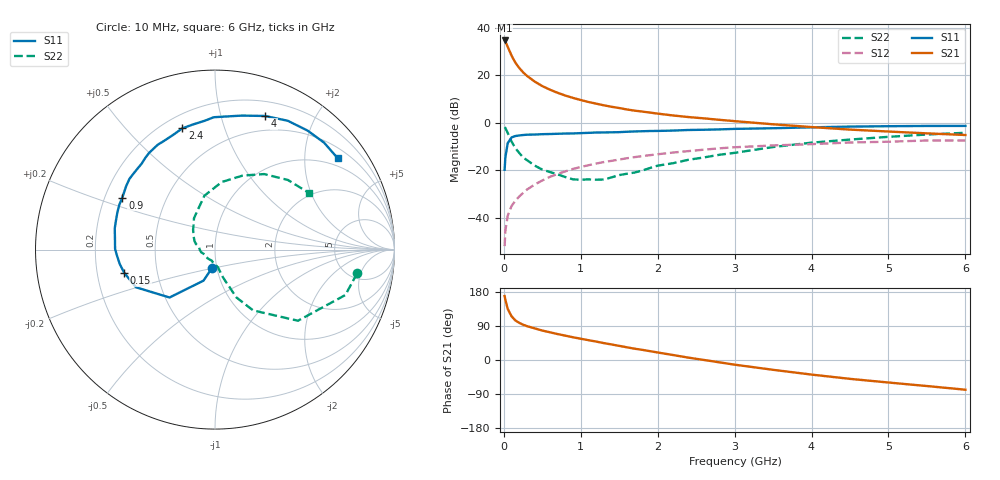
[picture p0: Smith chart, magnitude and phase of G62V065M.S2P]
! SIEMENS Small Signal Semiconductors
! BFG193
! Si NPN RF Bipolar Junction Transistor in SOT223
! VCE = 2 V  IC = 65 mA
! Common Emitter S-Parameters:  August  1996
# GHz  S  MA  R  50
!  f  S11  S21  S12  S22
! GHz  MAG  ANG  MAG  ANG  MAG  ANG  MAG  ANG
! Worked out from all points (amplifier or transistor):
!   36 points, 10 MHz to 6 GHz, reference 50 ohm
!   highest |S21| = 34.6 dB at 10 MHz (marker M1)
!   |S21| within 3 dB of that: start of sweep to 55.13 MHz
!   unconditionally stable (mu >= 1): start of sweep to 13.56 MHz; 234 MHz to 2.78 GHz
!   at 250 MHz: K = 1.02, MAG = 24.6 dB, |S12| = -29.6 dB
!   at 1.4 GHz: K = 1.09, MAG = 9.6 dB, |S12| = -16.1 dB
!   at 6 GHz: K = 0.97, MSG = 1.1 dB, |S12| = -7.5 dB
!   S11 on the Smith chart (normalised r, x): 10 MHz: 0.95, -0.19; 150 MHz: 0.32, -0.11; 900 MHz: 0.27, +0.24; 2.4 GHz: 0.28, +0.73; 4 GHz: 0.34, +1.39; 6 GHz: 0.76, +2.84
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0.01  0.1018 -98.6  53.74 168.8  0.0025 76.4  0.8026 -9.5
0.02  0.1848 -110.4  50.88 159.0  0.0053 75.8  0.7693 -19.2
0.05  0.3679 -133.5  39.77 135.1  0.0109 65.1  0.6089 -40.6
0.1  0.4878 -154.5  25.82 115.4  0.0175 64.1  0.4 -57.9
0.15  0.5219 -165.6  18.32 104.3  0.0227 64.6  0.2902 -66.1
0.2  0.5368 -171.4  14.21 98.1  0.0278 67.3  0.2297 -68.5
0.25  0.5479 -176.8  11.48 93.2  0.033 67.9  0.1854 -71.7
0.3  0.5567 179.6  9.672 89.4  0.0389 68.9  0.1622 -73.8
0.4  0.5608 173.7  7.328 83.5  0.0495 69.1  0.1248 -77.1
0.5  0.571 168.0  5.88 77.7  0.0605 68.1  0.1023 -79.9
0.6  0.5754 163.4  4.927 73.1  0.0722 66.9  0.091 -84.6
0.7  0.5823 159.0  4.24 68.4  0.083 65.6  0.0812 -91.7
0.9  0.5921 150.7  3.314 60.0  0.106 61.6  0.0638 -107.1
1.1  0.6089 144.3  2.718 52.3  0.1266 57.9  0.0638 -129.2
1.6  0.6424 127.1  1.892 33.5  0.1777 46.4  0.0838 -178.1
2.2  0.6798 110.2  1.414 13.1  0.2344 32.2  0.1397 148.4
2.4  0.6995 105.1  1.31 6.2  0.2513 27.8  0.1651 137.7
3.5  0.7614 78.7  0.922 -25.9  0.3306 -0.2  0.3061 101.1
4  0.7953 69.4  0.806 -38.5  0.3525 -10.1  0.3784 84.3
4.5  0.8245 60.5  0.713 -49.8  0.381 -20.4  0.4398 69.6
5.5  0.8511 44.4  0.594 -68.7  0.4201 -43.7  0.5615 43.7
6  0.8524 36.6  0.548 -78.4  0.4214 -57.0  0.6109 31.2
